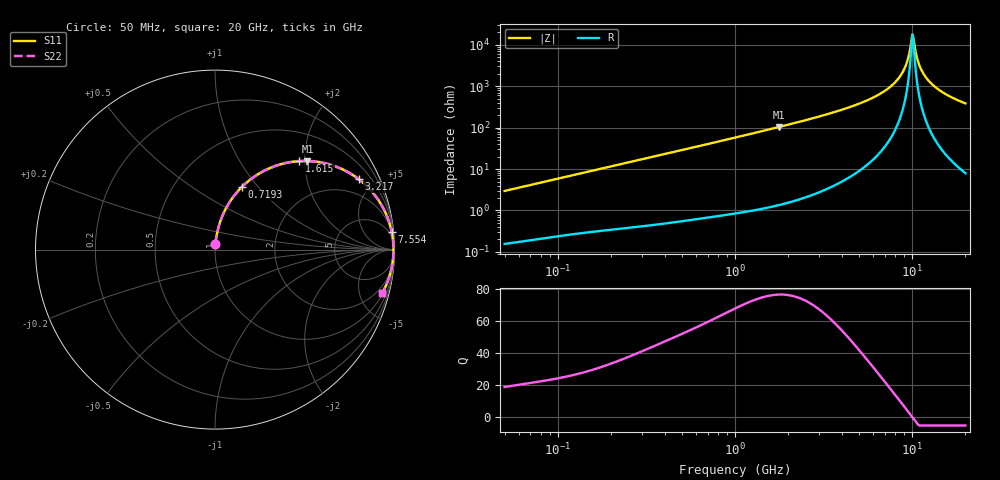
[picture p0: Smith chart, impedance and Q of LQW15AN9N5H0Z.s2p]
!Murata Part Number: LQW15AN9N5H0Z
!These Parameters are Measured in Series Mode Connection
!  o--[Z]--o
!Port1  Port2
!  o-------o
!Freq. Start=50[MHz] Stop=20[GHz], 401[Steps]
# Hz S RI R 50
!Freq.(Hz) S11(Real) S11(Imag) S21(Real) S21(Imag) S12(Real) S12(Imag) S22(Real) S22(Imag)
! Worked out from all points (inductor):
!   401 points, 50 MHz to 20 GHz, reference 50 ohm
!   read as one part in series: L = 9.37 nH near 51.52 MHz
!   highest Q = 76.6 at 1.767 GHz (marker M1), where L = 9.29 nH
!   self-resonance near 10.04 GHz
!   S11 on the Smith chart (normalised r, x): 50 MHz: 1.00, +0.06; 719.3 MHz: 1.01, +0.82; 1.615 GHz: 1.02, +1.88; 3.217 GHz: 1.06, +4.05; 7.554 GHz: 2, +19; 20 GHz: 1.16, -7.66
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5e7  0.00243 0.0295  0.9976 -0.0295  0.9976 -0.0295  0.00243 0.0295
1.364002e8  0.009 0.0781  0.991 -0.0781  0.991 -0.0781  0.009 0.0781
3.721004e8  0.0474 0.2019  0.9526 -0.2019  0.9526 -0.2019  0.0474 0.2019
7.192613e8  0.1485 0.3474  0.8515 -0.3474  0.8515 -0.3474  0.1485 0.3474
1e9  0.2501 0.4258  0.7499 -0.4258  0.7499 -0.4258  0.2501 0.4258
1.614971e9  0.4684 0.4925  0.5316 -0.4925  0.5316 -0.4925  0.4684 0.4925
1.766834e9  0.5151 0.4933  0.4849 -0.4933  0.4849 -0.4933  0.5151 0.4933
2.728004e9  0.7317 0.436  0.2683 -0.436  0.2683 -0.436  0.7317 0.436
3.216634e9  0.8001 0.3922  0.1999 -0.3922  0.1999 -0.3922  0.8001 0.3922
5.352748e9  0.9415 0.222  0.0585 -0.222  0.0585 -0.222  0.9415 0.222
7.442007e9  0.9829 0.1055  0.0171 -0.1055  0.0171 -0.1055  0.9829 0.1055
7.554318e9  0.9841 0.1002  0.0159 -0.1002  0.0159 -0.1002  0.9841 0.1002
8.907419e9  0.9925 0.0426  0.00745 -0.0426  0.00745 -0.0426  0.9925 0.0426
9.316812e9  0.9937 0.027  0.00633 -0.027  0.00633 -0.027  0.9937 0.027
9.892087e9  0.9944 0.00613  0.0056 -0.00613  0.0056 -0.00613  0.9944 0.00613
1.004137e10  0.9944 0.000918  0.00556 -0.000918  0.00556 -0.000918  0.9944 0.000918
1.034674e10  0.9944 -0.0095  0.00564 0.0095  0.00564 0.0095  0.9944 -0.0095
1.066139e10  0.9941 -0.0199  0.00593 0.0199  0.00593 0.0199  0.9941 -0.0199
1.115139e10  0.9932 -0.0356  0.00679 0.0356  0.00679 0.0356  0.9932 -0.0356
1.238412e10  0.9893 -0.0722  0.0107 0.0722  0.0107 0.0722  0.9893 -0.0722
1.504638e10  0.9743 -0.1406  0.0257 0.1406  0.0257 0.1406  0.9743 -0.1406
2e10  0.9319 -0.2417  0.0681 0.2417  0.0681 0.2417  0.9319 -0.2417
